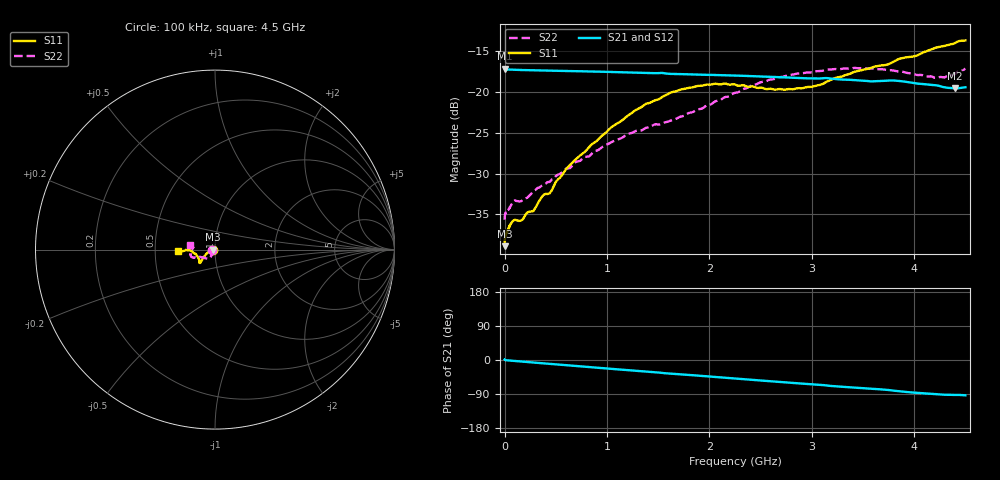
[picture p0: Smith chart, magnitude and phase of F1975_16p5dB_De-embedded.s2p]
! Integrated Device Technology
! Corporate Headquarters
! 6024 Silver Creek Valley Road
! San Jose, CA 95138  USA
! Phone:  1-408-284-8200
! Toll Free:  1-800-223-1366
! Webpage:  http://www.idt.com/
! Timing and RF Division
! 515 Groton Road, Suite 102
! Westford, MA 01886-6024
! Device:  F1975
! Description: 6-bit, 75 ohm, 0.5 dB Digital Step Attenuator
! Frequency:  5.0 MHz -  3.00 GHz
! Package:  4x4 mm QFN Plastic Package: 20 pin
! Ports:  2 RF, 11 DC
!  Pin  1  = D5 (16 dB)
!  Pin  2  = RF1  =  Port 1
!  Pin  3  = Serial Data In (DATA)
!  Pin  4  = Serial Clock (CLK)
!  Pin  5  = Serial Latch Enable (LE)
!  Pin  6  = VDD
!  Pin  7  = NC
!  Pin  8  = NC
!  Pin  9  = NC
!  Pin 10  = GND
!  Pin 11  = GND
!  Pin 12  = NC
!  Pin 13  = VMODE
!  Pin 14  = RF2  =  Port 2
!  Pin 15  = D4 (8 dB)
!  Pin 16  = D3 (4 dB)
!  Pin 17  = D2 (2 dB)
!  Pin 18  = NC
!  Pin 19  = D1 (1 dB)
!  Pin 20  = D0 (0.5 dB)
! State:  33
! Atten State:  16.5 dB
! Voltage:  +3.30 Volts
! Current:  0.561 mA
! Data:  The device was measured on a F1975 evaluation board which has
!  individual transmission lines to the RF pins.  Data was collected
!  using a calibrated network analyzer.  The evaluation board was
!  de-embedded using Automatic Fixture Removal (AFR).
!  The reference plane is the edge of the package pin.
! Misc:
!  Action Tracker AT0415
! Date Measured:  2018-02-08
! Date:  2018-03-26  MJV
! Note:
!  Integrated Device Technology supplies this data as a sample of measured
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# GHz S dB R 75
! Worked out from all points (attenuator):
!   291 points, 100 kHz to 4.5 GHz, reference 75 ohm
!   highest |S21| = -17.15 dB at 100 kHz (marker M1); lowest = -19.6 dB at 4.4 GHz (marker M2)
!   lowest |S11| = -38.9 dB at 100 kHz (marker M3), VSWR 1.02, Z = 73.3 + j0.0045 ohm
!   |S11| at or under -10 dB: start of sweep to end of sweep
!   |S22| runs from -35.7 to -17.0 dB; largest |S21 - S12| = 0.00015
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0.0001  -38.89 179.8  -17.15 1.2  -17.15 1.2  -35.65 -178.3
0.002  -38.07 -177.6  -17.19 0.8  -17.19 0.9  -35.18 -177.2
0.011  -37.56 -176.5  -17.22 -0.5  -17.22 -0.4  -34.75 -175.2
0.08  -35.81 -170.6  -17.26 -2.1  -17.26 -2.1  -33.47 -165.3
0.16  -35.76 -168.0  -17.30 -4.0  -17.30 -4.0  -33.39 -152.4
0.22  -34.77 -169.2  -17.31 -5.3  -17.31 -5.3  -32.96 -145.9
0.28  -34.59 -168.2  -17.33 -6.6  -17.33 -6.6  -32.17 -142.4
0.38  -32.61 -166.5  -17.36 -8.9  -17.36 -8.9  -31.44 -133.2
0.44  -32.42 -165.7  -17.37 -10.1  -17.37 -10.1  -31.02 -128.6
0.6  -29.44 -163.2  -17.42 -13.7  -17.42 -13.7  -29.40 -124.0
0.76  -27.56 -157.1  -17.46 -17.2  -17.45 -17.2  -28.15 -121.7
1.06  -24.16 -150.5  -17.54 -23.7  -17.54 -23.7  -26.04 -119.9
1.52  -20.78 -141.5  -17.66 -33.5  -17.66 -33.5  -23.97 -129.0
1.88  -19.26 -138.4  -17.86 -41.1  -17.85 -41.1  -22.15 -143.9
2.26  -19.13 -140.2  -17.98 -49.0  -17.98 -49.0  -20.07 -155.0
2.64  -19.71 -150.5  -18.15 -56.9  -18.15 -56.9  -18.37 -158.2
3.02  -19.29 -165.7  -18.32 -64.5  -18.32 -64.5  -17.52 -160.9
3.42  -17.51 -176.5  -18.53 -73.2  -18.53 -73.2  -17.04 -166.9
3.76  -16.53 -178.4  -18.58 -79.5  -18.58 -79.5  -17.33 -173.5
4.2  -14.61 -177.2  -19.15 -89.9  -19.15 -89.9  -18.25 175.0
4.4  -13.98 -176.3  -19.55 -92.2  -19.55 -92.2  -17.80 171.9
4.5  -13.67 -178.2  -19.41 -93.3  -19.41 -93.3  -17.12 170.5
